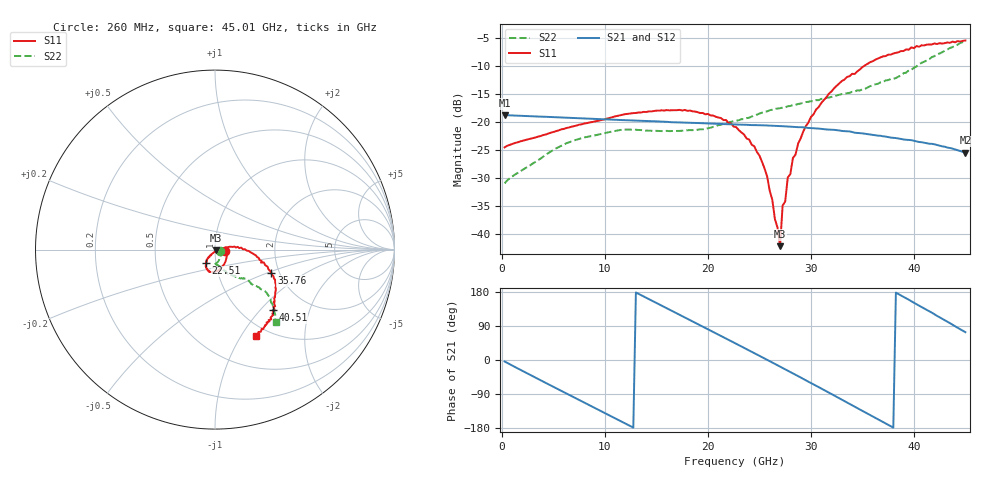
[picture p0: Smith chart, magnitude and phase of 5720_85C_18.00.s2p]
! Device:  ADRF5720
! Description: 0.5dB LSB GaAs MMIC 6-bit Digital Attenuator
! Frequency:  0.000009 -  40 GHz
! Ports:
!	RF1	= Port 1
!	RF2	= Port 2
! Vdd:  3.3 Volt
! Vss:  -3.3 Volt
! Control:  0/3.3 Volt
! State:  18.00 dB attenuation
! Data:  The device was measured using G-S-G Probes on a matrix board.
!  Data was collected using an calibrated 4 port network analyzer.
!  The reference plane for this measurement is at the launchers.
! Note:  Analog Devices supplies this data as a sample of measured data
!  for this product.  Your particular data for this product may vary.
!  Data was taken at 85 degrees C.
!  Analog Devices reserves the right to change this data at anytime.
# GHZ S DB R 45.0
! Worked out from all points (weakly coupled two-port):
!   180 points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, 260 MHz to 45.01 GHz, reference 45 ohm
!   highest |S21| = -18.84 dB at 260 MHz (marker M1); lowest = -25.6 dB at 45.01 GHz (marker M2)
!   lowest |S11| = -42.2 dB at 27.01 GHz (marker M3), VSWR 1.02, Z = 45.6 - j0.395 ohm
!   |S11| at or under -10 dB: start of sweep to 35.22 GHz
!   |S22| runs from -31.0 to -5.6 dB; largest |S21 - S12| = 0.00058
!   S11 on the Smith chart (normalised r, x): 260 MHz: 1.12, -0.02; 22.51 GHz: 0.90, -0.14; 35.76 GHz: 1.81, -0.53; 40.51 GHz: 1.36, -1.18; 45.01 GHz: 0.86, -1.16
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0.26  -24.60 -9.0  -18.84 -3.9  -18.84 -3.9  -31.04 -17.4
7.76  -20.48 -56.7  -19.41 -109.2  -19.40 -109.1  -22.94 -77.9
15.26  -18.04 -94.5  -19.97 146.8  -19.96 147.0  -21.66 -93.9
20.01  -18.62 -113.2  -20.32 81.0  -20.30 81.2  -21.18 -80.2
22.51  -20.89 -123.2  -20.50 46.1  -20.48 46.3  -19.92 -72.0
22.76  -21.01 -122.8  -20.51 42.7  -20.50 42.9  -19.83 -72.2
24.51  -24.42 -128.4  -20.62 18.3  -20.61 18.5  -18.93 -69.4
25.51  -28.40 -124.0  -20.67 4.0  -20.65 4.3  -18.21 -68.0
26.26  -33.98 -116.6  -20.73 -6.7  -20.72 -6.5  -17.87 -66.0
27.01  -42.25 -34.2  -20.78 -17.5  -20.77 -17.2  -17.60 -64.2
27.26  -34.99 -10.3  -20.82 -21.1  -20.81 -20.9  -17.50 -64.6
27.51  -34.26 6.5  -20.85 -24.6  -20.84 -24.4  -17.45 -63.5
27.76  -29.99 5.7  -20.88 -28.2  -20.86 -27.9  -17.25 -64.2
28.01  -29.36 10.0  -20.91 -31.9  -20.90 -31.6  -17.21 -63.6
28.26  -26.50 9.9  -20.94 -35.3  -20.92 -35.1  -17.04 -64.0
28.76  -23.95 11.5  -20.99 -42.4  -20.97 -42.2  -16.86 -63.3
30.26  -18.70 5.8  -21.18 -64.3  -21.16 -64.0  -16.38 -61.4
33.01  -12.75 -8.2  -21.66 -104.8  -21.64 -104.6  -15.07 -55.8
35.76  -9.38 -22.5  -22.30 -145.4  -22.28 -145.1  -13.66 -49.9
37.76  -8.03 -31.8  -22.85 -174.9  -22.83 -174.6  -12.39 -43.6
40.51  -6.63 -46.5  -23.64 143.5  -23.62 143.9  -9.72 -40.6
45.01  -5.50 -64.8  -25.55 73.4  -25.51 73.7  -5.56 -50.0
